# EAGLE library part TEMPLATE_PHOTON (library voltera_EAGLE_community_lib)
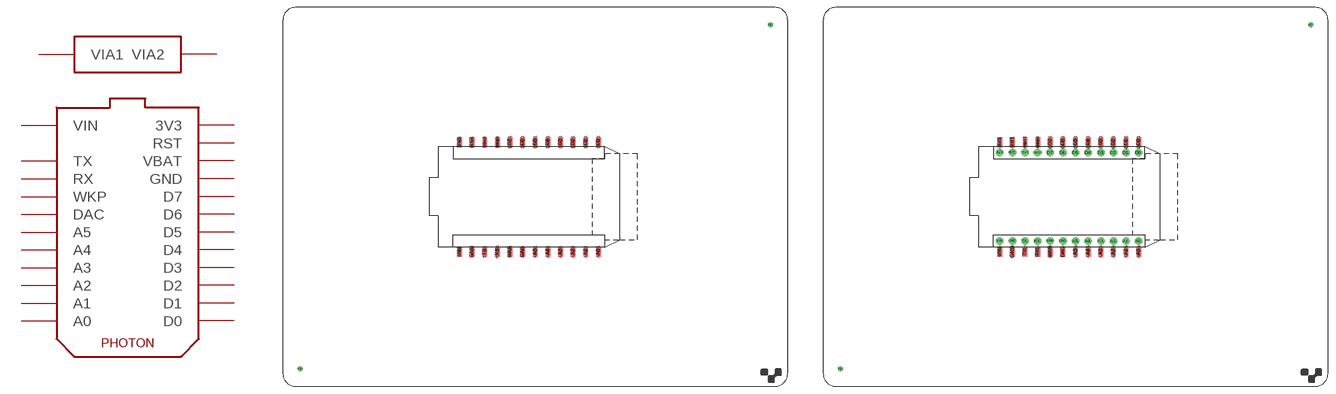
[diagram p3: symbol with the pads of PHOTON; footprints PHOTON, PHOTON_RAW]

Designator prefix -

## TEMPLATE_PHOTON_SHIELD  [PHOTON]
3V3  3V3
3V3@1  3V3
A0  A0
A0@1  A0
A1  A1
A1@1  A1
A2  A2
A2@1  A2
A3  A3
A3@1  A3
A4  A4
A4@1  A4
A5  A5
A5@1  A5
D0  D0
D0@1  D0
D1  D1
D1@1  D1
D2  D2
D2@1  D2
D3  D3
D3@1  D3
D4  D4
D4@1  D4
D5  D5
D5@1  D5
D6  D6
D6@1  D6
D7  D7
D7@1  D7
DAC  DAC
DAC@1  DAC
GND  GND
GND@1  GND
GND@2  GND
GND@3  GND
P$1  VIA1
P$2  VIA2
RST  RST
RST@1  RST
RX  RX
RX@1  RX
TX  TX
TX@1  TX
VBAT  VBAT
VBAT@1  VBAT
VIN  VIN
VIN@1  VIN
WKP  WKP
WKP@1  WKP

## TEMPLATE_PHOTON_RAW  [PHOTON_RAW]
3V3  3V3
3V3.  3V3
3V31  3V3
A0  A0
A0.  A0
A0@1  A0
A1  A1
A1.  A1
A1@1  A1
A2  A2
A2.  A2
A2@1  A2
A3  A3
A3.  A3
A3@1  A3
A4  A4
A4.  A4
A4@1  A4
A5  A5
A5.  A5
A5@1  A5
D0  D0
D0.  D0
D0@1  D0
D1  D1
D1.  D1
D1@1  D1
D2  D2
D2.  D2
D2@1  D2
D3  D3
D3.  D3
D3@1  D3
D4  D4
D4.  D4
D4@1  D4
D5  D5
D5.  D5
D5@1  D5
D6  D6
D6.  D6
D6@1  D6
D7  D7
D7.  D7
D7@1  D7
DAC  DAC
DAC1  DAC
DAC.  DAC
GND  GND
GND1  GND
GND.  GND
GND.@1  GND
GND@1  GND
GND@2  GND
P$1  VIA1
P$2  VIA2
RST  RST
RST1  RST
RST.  RST
RX  RX
RX1  RX
RX.  RX
TX  TX
TX1  TX
TX.  TX
VBAT  VBAT
VBAT1  VBAT
VBAT.  VBAT
VIN  VIN
VIN1  VIN
VIN.  VIN
WKP  WKP
WKP1  WKP
WKP.  WKP

## Footprint PHOTON (pad centres in mm)
smd 1 x 2 bottom: 3V3 35.56,49.13; A0 63.5,27.07; A1 60.96,27.07; A2 58.42,27.07; A3 55.88,27.07; A4 53.34,27.07; A5 50.8,27.07; D0 63.5,49.13; D1 60.96,49.13; D2 58.42,49.13; D3 55.88,49.13; D4 53.34,49.13; D5 50.8,49.13; D6 48.26,49.13; D7 45.72,49.13; DAC 48.26,27.07; GND 38.1,27.07; GND@1 43.18,49.13; RST 38.1,49.13; RX 43.18,27.07; TX 40.64,27.07; VBAT 40.64,49.13; VIN 35.56,27.07; WKP 45.72,27.07
smd 1 x 2: 3V3@1 35.56,49.13; A0@1 63.5,27.07; A1@1 60.96,27.07; A2@1 58.42,27.07; A3@1 55.88,27.07; A4@1 53.34,27.07; A5@1 50.8,27.07; D0@1 63.5,49.13; D1@1 60.96,49.13; D2@1 58.42,49.13; D3@1 55.88,49.13; D4@1 53.34,49.13; D5@1 50.8,49.13; D6@1 48.26,49.13; D7@1 45.72,49.13; DAC@1 48.26,27.07; GND@2 43.18,49.13; GND@3 38.1,27.07; RST@1 38.1,49.13; RX@1 43.18,27.07; TX@1 40.64,27.07; VBAT@1 40.64,49.13; VIN@1 35.56,27.07; WKP@1 45.72,27.07
drill 0.3 pad 1: P$1 3.5,3.5; P$2 98.1,72.7

## Footprint PHOTON_RAW (pad centres in mm)
smd 1 x 2 bottom: 3V3 35.56,49.13; A0 63.5,27.07; A1 60.96,27.07; A2 58.42,27.07; A3 55.88,27.07; A4 53.34,27.07; A5 50.8,27.07; D0 63.5,49.13; D1 60.96,49.13; D2 58.42,49.13; D3 55.88,49.13; D4 53.34,49.13; D5 50.8,49.13; D6 48.26,49.13; D7 45.72,49.13; DAC 48.26,27.07; GND 38.1,27.07; GND@1 43.18,49.13; RST 38.1,49.13; RX 43.18,27.07; TX 40.64,27.07; VBAT 40.64,49.13; VIN 35.56,27.07; WKP 45.72,27.07
drill 1: 3V3. 35.56,46.99; A0. 63.5,29.21; A1. 60.96,29.21; A2. 58.42,29.21; A3. 55.88,29.21; A4. 53.34,29.21; A5. 50.8,29.21; D0. 63.5,46.99; D1. 60.96,46.99; D2. 58.42,46.99; D3. 55.88,46.99; D4. 53.34,46.99; D5. 50.8,46.99; D6. 48.26,46.99; D7. 45.72,46.99; DAC. 48.26,29.21; GND. 38.1,29.21; GND.@1 43.18,46.99; RST. 38.1,46.99; RX. 43.18,29.21; TX. 40.64,29.21; VBAT. 40.64,46.99; VIN. 35.56,29.21; WKP. 45.72,29.21
smd 1 x 2: 3V31 35.56,49.13; A0@1 63.5,27.07; A1@1 60.96,27.07; A2@1 58.42,27.07; A3@1 55.88,27.07; A4@1 53.34,27.07; A5@1 50.8,27.07; D0@1 63.5,49.13; D1@1 60.96,49.13; D2@1 58.42,49.13; D3@1 55.88,49.13; D4@1 53.34,49.13; D5@1 50.8,49.13; D6@1 48.26,49.13; D7@1 45.72,49.13; DAC1 48.26,27.07; GND1 38.1,27.07; GND@2 43.18,49.13; RST1 38.1,49.13; RX1 43.18,27.07; TX1 40.64,27.07; VBAT1 40.64,49.13; VIN1 35.56,27.07; WKP1 45.72,27.07
drill 0.3 pad 1: P$1 3.5,3.5; P$2 98.1,72.7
